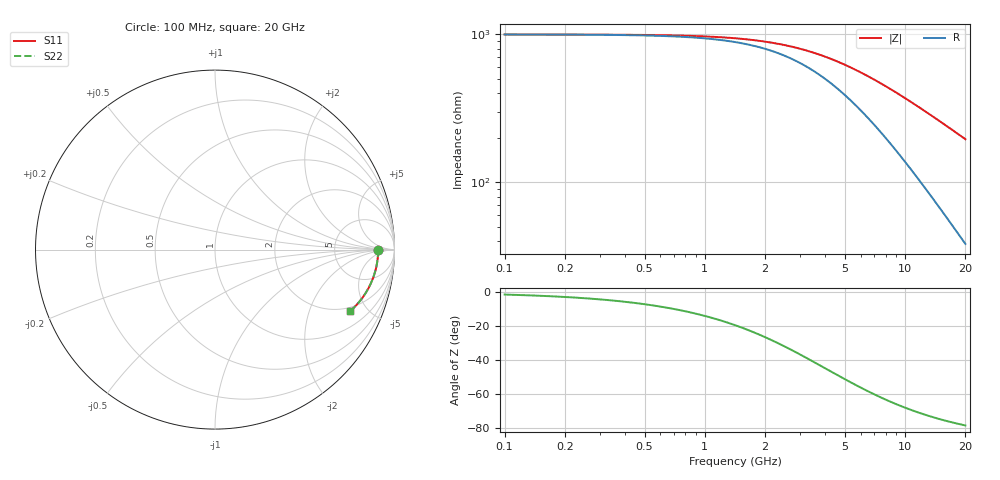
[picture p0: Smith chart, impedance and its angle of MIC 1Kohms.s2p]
! Vishay ElectroFilms Inc.
! MIC001 10000 - 1K Ohm in Series Configuration
! March 2012
# GHz S MA R 50
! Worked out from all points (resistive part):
!   233 points, 100 MHz to 20 GHz, reference 50 ohm
!   read as one part in series: R = 999 ohm at 102.3 MHz
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0.1  0.9091 -0.1  0.09094 1.3  0.09094 1.3  0.9091 -0.1
0.2436751  0.9091 -0.3  0.09108 3.2  0.09108 3.2  0.9091 -0.3
0.5937753  0.909 -0.8  0.0919 7.7  0.0919 7.7  0.909 -0.8
0.9591909  0.9089 -1.3  0.09347 12.3  0.09347 12.3  0.9089 -1.3
1.178065  0.9088 -1.5  0.09475 14.9  0.09475 14.9  0.9088 -1.5
1.414214  0.9086 -1.8  0.09639 17.7  0.09639 17.7  0.9086 -1.8
1.818091  0.9083 -2.4  0.0998 22.1  0.0998 22.1  0.9083 -2.4
2.284535  0.9079 -3.0  0.1046 26.8  0.1046 26.8  0.9079 -3.0
2.805834  0.9072 -3.7  0.1109 31.4  0.1109 31.4  0.9072 -3.7
3.446086  0.9063 -4.5  0.1197 36.3  0.1197 36.3  0.9063 -4.5
4.232434  0.9049 -5.5  0.1318 41.2  0.1318 41.2  0.9049 -5.5
5.198215  0.9028 -6.7  0.1482 45.7  0.1482 45.7  0.9028 -6.7
5.827005  0.9012 -7.6  0.1594 48.0  0.1594 48.0  0.9012 -7.6
6.531856  0.8992 -8.5  0.1724 50.1  0.1724 50.1  0.8992 -8.5
8.397251  0.8929 -10.8  0.2079 53.7  0.2079 53.7  0.8929 -10.8
10.79537  0.8828 -13.8  0.2544 55.9  0.2544 55.9  0.8828 -13.8
12.10121  0.8765 -15.4  0.2796 56.3  0.2796 56.3  0.8765 -15.4
13.56501  0.8686 -17.2  0.3075 56.4  0.3075 56.4  0.8686 -17.2
15.20587  0.8591 -19.1  0.3382 56.2  0.3382 56.2  0.8591 -19.1
16.66035  0.85 -20.8  0.3646 55.8  0.3646 55.8  0.85 -20.8
18.25396  0.8395 -22.6  0.3928 55.1  0.3928 55.1  0.8395 -22.6
20  0.8274 -24.5  0.4225 54.2  0.4225 54.2  0.8274 -24.5
